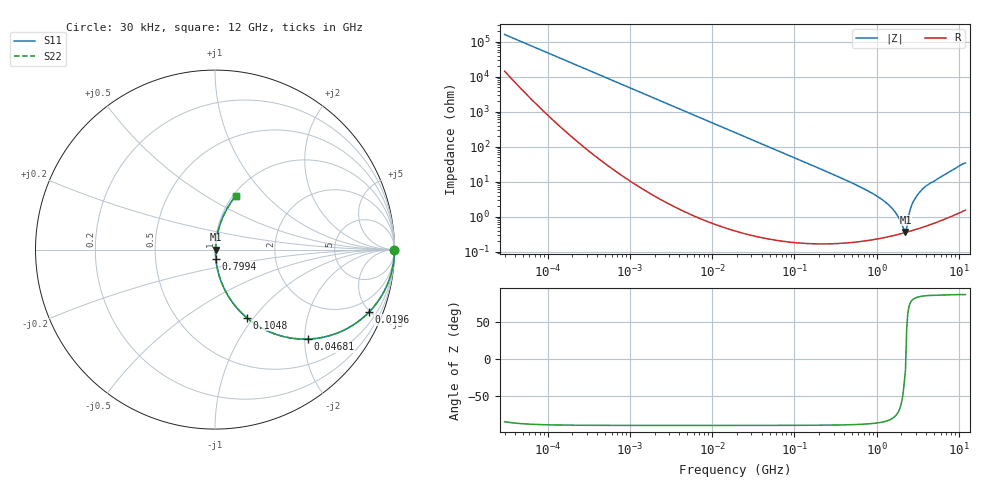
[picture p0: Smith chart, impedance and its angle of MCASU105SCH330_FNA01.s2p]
! MCASU105SCH330_FNA01  S-PARAMETER MODEL  ( General Type )
! Model Generated by TAIYO YUDEN Corporation (http://www.ty-top.com)
! Version 1.0
! TAIYO YUDEN Control No. 130207
! Copyright(c) 2013 TAIYO YUDEN CO.,LTD. All Rights Reserved.
! Product Description (link to TY-COMPAS)
! https://ds.yuden.co.jp/TYCOMPAS/or/detail?pn=MCASU105SCH330JFNA01&u=M
! Products Name : Multilayer Ceramic Capacitors
! Characteristics :
!  Capacitance : 33 pF , Rated Voltage : 50V , TCC : CH / C0H
!  Case Size : 1.0 x 0.5 / 0.039 x 0.02 [mm/inch] , Thickness : 0.5 / 0.02 [mm/inch]
!  (Conditions: Temperature = 25 degC , DC Bias Current/Voltage = 0A / 0V)
! External Node Assignments :
!  1  o---| |---o  2
! GND o---------o GND
! Frequency Range : 30000Hz  -  12GHz  [ 401 STEP ]
# MHz S RI R 50
! Freq[MHz].  S11 Real  S11 Imag  S21 Real  S21 Imag  S12 Real  S12 Imag  S22 Real  S22 Imag
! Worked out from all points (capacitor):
!   401 points, 30 kHz to 12 GHz, reference 50 ohm
!   read as one part in series: C = 32.9 pF near 32 kHz
!   lowest |Z| = 362 mohm at 2.243 GHz (marker M1)
!   series resonance near 2.26 GHz, so ESL is about 150 pH
!   S11 on the Smith chart (normalised r, x): 30 kHz: open; 19.6 MHz: 1.01, -4.93; 46.81 MHz: 1.00, -2.06; 104.8 MHz: 1.00, -0.92; 799.4 MHz: 1.00, -0.11; 12 GHz: 1.03, +0.68
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0.03  0.9999 -0.000616  5.53e-05 0.000616  5.53e-05 0.000616  0.9999 -0.000616
0.260295  0.9999 -0.00538  6.06e-05 0.00538  6.06e-05 0.00538  0.9999 -0.00538
2.258455  0.9978 -0.0466  0.00225 0.0466  0.00225 0.0466  0.9978 -0.0466
7.211021  0.978 -0.1459  0.022 0.1459  0.022 0.1459  0.978 -0.1459
18.97367  0.8661 -0.3398  0.1339 0.3398  0.1339 0.3398  0.8661 -0.3398
19.5955  0.8584 -0.3478  0.1416 0.3478  0.1416 0.3478  0.8584 -0.3478
46.80535  0.5158 -0.4986  0.4842 0.4986  0.4842 0.4986  0.5158 -0.4986
104.8152  0.1757 -0.3786  0.8243 0.3786  0.8243 0.3786  0.1757 -0.3786
164.6252  0.0799 -0.2683  0.9201 0.2683  0.9201 0.2683  0.0799 -0.2683
345.6326  0.0199 -0.1337  0.9801 0.1337  0.9801 0.1337  0.0199 -0.1337
799.3715  0.00487 -0.0527  0.9951 0.0527  0.9951 0.0527  0.00487 -0.0527
1428.372  0.00311 -0.0204  0.9969 0.0204  0.9969 0.0204  0.00311 -0.0204
1790.1  0.00315 -0.0103  0.9968 0.0103  0.9968 0.0103  0.00315 -0.0103
2103.309  0.00337 -0.00338  0.9966 0.00338  0.9966 0.00338  0.00337 -0.00338
2243.435  0.0035 -0.00089  0.9965 0.00089  0.9965 0.00089  0.0035 -0.00089
2316.96  0.00358 0.00295  0.9964 -0.00295  0.9964 -0.00295  0.00358 0.00295
2552.314  0.00403 0.0149  0.996 -0.0149  0.996 -0.0149  0.00403 0.0149
2722.352  0.00453 0.0234  0.9955 -0.0234  0.9955 -0.0234  0.00453 0.0234
2998.885  0.0055 0.0351  0.9945 -0.0351  0.9945 -0.0351  0.0055 0.0351
3523.591  0.00809 0.0571  0.9919 -0.0571  0.9919 -0.0571  0.00809 0.0571
6502.545  0.0303 0.1468  0.9697 -0.1468  0.9697 -0.1468  0.0303 0.1468
12000  0.1151 0.2976  0.8849 -0.2976  0.8849 -0.2976  0.1151 0.2976
